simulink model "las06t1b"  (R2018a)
settings: Solver=ode45  StartTime=0.0  StopTime=10  MaxStep=10  MinStep=0.0001  RelTol=1e-3  AbsTol=1e-3  EnableMultiTasking=on

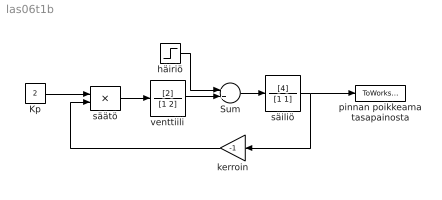
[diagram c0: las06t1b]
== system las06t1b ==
  Kp : Constant  Value=2
  Sum : Sum
  häiriö : Step  Time=3  After=-1
  kerroin : Gain  Gain=-1
  pinnan poikkeama tasapainosta : ToWorkspace  VariableName=y
  säiliö : TransferFcn  Numerator=[4]  Denominator=[1 1]
  säätö : Product
  venttiili : TransferFcn  Numerator=[2]  Denominator=[1 2]
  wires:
  häiriö/1 -> Sum/1
  venttiili/1 -> Sum/2
  Sum/1 -> säiliö/1
  säiliö/1 -> pinnan poikkeama tasapainosta/1, kerroin/1
  säätö/1 -> venttiili/1
  Kp/1 -> säätö/1
  kerroin/1 -> säätö/2
